PROGRAM P_Prog3
VAR

	fbKL6401 					: FB_LON_KL6401;

	fbREAD_063		: FB_READ_063_SNVT_temp_f;
	fbSEND_063		: FB_SEND_063_SNVT_temp_f;

	fbREAD_064		: FB_READ_064_SNVT_time_f;
	fbSEND_064		: FB_SEND_064_SNVT_time_f;

	fbREAD_065		: FB_READ_065_SNVT_vol_f;
	fbSEND_065		: FB_SEND_065_SNVT_vol_f;

	fbREAD_066		: FB_READ_066_SNVT_volt_f;
	fbSEND_066		: FB_SEND_066_SNVT_volt_f;

	fbREAD_067		: FB_READ_067_SNVT_btu_f;
	fbSEND_067		: FB_SEND_067_SNVT_btu_f;

	fbREAD_068		: FB_READ_068_SNVT_elec_whr_f;
	fbSEND_068		: FB_SEND_068_SNVT_elec_whr_f;

	fbREAD_069		: FB_READ_069_SNVT_config_src;
	fbSEND_069		: FB_SEND_069_SNVT_config_src;

	fbREAD_070		: FB_READ_070_SNVT_color;
	fbSEND_070		: FB_SEND_070_SNVT_color;

	fbREAD_071		: FB_READ_071_SNVT_grammage;
	fbSEND_071		: FB_SEND_071_SNVT_grammage;

	fbREAD_072		: FB_READ_072_SNVT_grammage_f;
	fbSEND_072		: FB_SEND_072_SNVT_grammage_f;

	fbREAD_073		: FB_READ_073_SNVT_file_req;
	fbSEND_073		: FB_SEND_073_SNVT_file_req;

	fbREAD_074		: FB_READ_074_SNVT_file_status;
	fbSEND_074		: FB_SEND_074_SNVT_file_status;

	fbREAD_075		: FB_READ_075_SNVT_freq_f;
	fbSEND_075		: FB_SEND_075_SNVT_freq_f;

	fbREAD_076		: FB_READ_076_SNVT_freq_hz;
	fbSEND_076		: FB_SEND_076_SNVT_freq_hz;

	fbREAD_077		: FB_READ_077_SNVT_freq_kilohz;
	fbSEND_077		: FB_SEND_077_SNVT_freq_kilohz;

	fbREAD_078		: FB_READ_078_SNVT_freq_milhz;
	fbSEND_078		: FB_SEND_078_SNVT_freq_milhz;

	fbREAD_079		: FB_READ_079_SNVT_lux;
	fbSEND_079		: FB_SEND_079_SNVT_lux;
(*
	fbREAD_080		: FB_READ_080;
	fbSEND_080		: FB_SEND_080_SNVT_angle_vel_f;
*)
	fbREAD_081		: FB_READ_081_SNVT_lev_percent;
	fbSEND_081		: FB_SEND_081_SNVT_lev_percent;

	fbREAD_082		: FB_READ_082_SNVT_multiplier;
	fbSEND_082		: FB_SEND_082_SNVT_multiplier;

	fbREAD_083		: FB_READ_083_SNVT_state;
	fbSEND_083		: FB_SEND_083_SNVT_state;

	fbREAD_084		: FB_READ_084_SNVT_time_stamp;
	fbSEND_084		: FB_SEND_084_SNVT_time_stamp;

	fbREAD_085		: FB_READ_085_SNVT_zerospan;
	fbSEND_085		: FB_SEND_085_SNVT_zerospan;

	fbREAD_086		: FB_READ_086_SNVT_magcard;
	fbSEND_086		: FB_SEND_086_SNVT_magcard;

	fbREAD_087		: FB_READ_087_SNVT_elapsed_tm;
	fbSEND_087		: FB_SEND_087_SNVT_elapsed_tm;

	fbREAD_088		: FB_READ_088_SNVT_alarm;
	fbSEND_088		: FB_SEND_088_SNVT_alarm;

	fbREAD_089		: FB_READ_089_SNVT_currency;
	fbSEND_089		: FB_SEND_089_SNVT_currency;

	fbREAD_090		: FB_READ_090_SNVT_file_pos;
	fbSEND_090		: FB_SEND_090_SNVT_file_pos;

	fbREAD_091		: FB_READ_091_SNVT_muldiv;
	fbSEND_091		: FB_SEND_091_SNVT_muldiv;

	fbREAD_092		: FB_READ_092_SNVT_obj_request;
	fbSEND_092		: FB_SEND_092_SNVT_obj_request;

	fbREAD_093		: FB_READ_093_SNVT_obj_status;
	fbSEND_093		: FB_SEND_093_SNVT_obj_status;

END_VAR


fbKL6401(
	bDisabled:=FALSE ,
	stParameter_IN:=LON_IN_3 ,
	stParameter_OUT:=LON_OUT_3 ,
	stLON_Com:=stLON_Com_3,
	bReady=> ,
	eError=> ,
	stKL6401=> ,
	arrProgID=> ,
	arrNeuronID=> ,
	bBusy=> ,
	bError=> ,
	dwErrorKL=> ,
	bTimeOut=> ,
	byLONState=> );

(**)
fbREAD_063(
	wNVIndex:=0 ,
	bDisabled:= ,
	stLON_Com:=stLON_Com_3,
	rValue=> ,
	bNewData=> ,
	bError=> ,
	eError=> );
fbREAD_063.rValue;
fbREAD_063.bError;
fbREAD_063.eError;

fbSEND_063.rValue;
fbSEND_063.bStart;
fbSEND_063.bError;
fbSEND_063.eError;
fbSEND_063.bBusy;
fbSEND_063.dwErrorKL;

fbSEND_063.bAuto;
fbSEND_063.bSendInit;
fbSEND_063.tMinSendTime;
fbSEND_063.tMaxSendTime;
fbSEND_063.rValueLimit;

fbSEND_063(
	wNVIndex:=1 ,
	bStart:= ,
	rValue:= ,
	bDisabled:= ,
	stLON_Com:=stLON_Com_3,
	bError=> ,
	eError=> );
fbSEND_063.bStart:=FALSE;

(**)
fbREAD_064(
	wNVIndex:=2 ,
	bDisabled:= ,
	stLON_Com:=stLON_Com_3,
	rValue=> ,
	bNewData=> ,
	bError=> ,
	eError=> );
fbREAD_064.rValue;
fbREAD_064.bError;
fbREAD_064.eError;

fbSEND_064.rValue;
fbSEND_064.bStart;
fbSEND_064.bError;
fbSEND_064.eError;
fbSEND_064.bBusy;
fbSEND_064.dwErrorKL;

fbSEND_064.bAuto;
fbSEND_064.bSendInit;
fbSEND_064.tMinSendTime;
fbSEND_064.tMaxSendTime;
fbSEND_064.rValueLimit;

fbSEND_064(
	wNVIndex:=3 ,
	bStart:= ,
	rValue:= ,
	bDisabled:= ,
	stLON_Com:=stLON_Com_3,
	bError=> ,
	eError=> );
fbSEND_064.bStart:=FALSE;

(**)
fbREAD_065(
	wNVIndex:=4 ,
	bDisabled:= ,
	stLON_Com:=stLON_Com_3,
	rValue=> ,
	bNewData=> ,
	bError=> ,
	eError=> );
fbREAD_065.rValue;
fbREAD_065.bError;
fbREAD_065.eError;

fbSEND_065.rValue;
fbSEND_065.bStart;
fbSEND_065.bError;
fbSEND_065.eError;
fbSEND_065.bBusy;
fbSEND_065.dwErrorKL;

fbSEND_065.bAuto;
fbSEND_065.bSendInit;
fbSEND_065.tMinSendTime;
fbSEND_065.tMaxSendTime;
fbSEND_065.rValueLimit;

fbSEND_065(
	wNVIndex:=5 ,
	bStart:= ,
	rValue:= ,
	bDisabled:= ,
	stLON_Com:=stLON_Com_3,
	bError=> ,
	eError=> );
fbSEND_065.bStart:=FALSE;

(**)
fbREAD_066(
	wNVIndex:=6 ,
	bDisabled:= ,
	stLON_Com:=stLON_Com_3,
	rValue=> ,
	bNewData=> ,
	bError=> ,
	eError=> );
fbREAD_066.rValue;
fbREAD_066.bError;
fbREAD_066.eError;

fbSEND_066.rValue;
fbSEND_066.bStart;
fbSEND_066.bError;
fbSEND_066.eError;
fbSEND_066.bBusy;
fbSEND_066.dwErrorKL;

fbSEND_066.bAuto;
fbSEND_066.bSendInit;
fbSEND_066.tMinSendTime;
fbSEND_066.tMaxSendTime;
fbSEND_066.rValueLimit;

fbSEND_066(
	wNVIndex:=7 ,
	bStart:= ,
	rValue:= ,
	bDisabled:= ,
	stLON_Com:=stLON_Com_3,
	bError=> ,
	eError=> );
fbSEND_066.bStart:=FALSE;

(**)
fbREAD_067(
	wNVIndex:=8 ,
	bDisabled:= ,
	stLON_Com:=stLON_Com_3,
	rValue=> ,
	bNewData=> ,
	bError=> ,
	eError=> );
fbREAD_067.rValue;
fbREAD_067.bError;
fbREAD_067.eError;

fbSEND_067.rValue;
fbSEND_067.bStart;
fbSEND_067.bError;
fbSEND_067.eError;
fbSEND_067.bBusy;
fbSEND_067.dwErrorKL;

fbSEND_067.bAuto;
fbSEND_067.bSendInit;
fbSEND_067.tMinSendTime;
fbSEND_067.tMaxSendTime;
fbSEND_067.rValueLimit;

fbSEND_067(
	wNVIndex:=9 ,
	bStart:= ,
	rValue:= ,
	bDisabled:= ,
	stLON_Com:=stLON_Com_3,
	bError=> ,
	eError=> );
fbSEND_067.bStart:=FALSE;

(**)
fbREAD_068(
	wNVIndex:=10 ,
	bDisabled:= ,
	stLON_Com:=stLON_Com_3,
	rValue=> ,
	bNewData=> ,
	bError=> ,
	eError=> );
fbREAD_068.rValue;
fbREAD_068.bError;
fbREAD_068.eError;

fbSEND_068.rValue;
fbSEND_068.bStart;
fbSEND_068.bError;
fbSEND_068.eError;
fbSEND_068.bBusy;
fbSEND_068.dwErrorKL;

fbSEND_068.bAuto;
fbSEND_068.bSendInit;
fbSEND_068.tMinSendTime;
fbSEND_068.tMaxSendTime;
fbSEND_068.rValueLimit;

fbSEND_068(
	wNVIndex:=11 ,
	bStart:= ,
	rValue:= ,
	bDisabled:= ,
	stLON_Com:=stLON_Com_3,
	bError=> ,
	eError=> );
fbSEND_068.bStart:=FALSE;

(**)
fbREAD_069(
	wNVIndex:=12 ,
	bDisabled:= ,
	stLON_Com:=stLON_Com_3,
	eValue=> ,
	bNewData=> ,
	bError=> ,
	eError=> );
fbREAD_069.eValue;
fbREAD_069.bError;
fbREAD_069.eError;

fbSEND_069.eValue;
fbSEND_069.bStart;
fbSEND_069.bError;
fbSEND_069.eError;
fbSEND_069.bBusy;
fbSEND_069.dwErrorKL;

fbSEND_069.bAuto;
fbSEND_069.bSendInit;
fbSEND_069.tMinSendTime;
fbSEND_069.tMaxSendTime;

fbSEND_069(
	wNVIndex:=13 ,
	bStart:= ,
	eValue:= ,
	bDisabled:= ,
	stLON_Com:=stLON_Com_3,
	bError=> ,
	eError=> );
fbSEND_069.bStart:=FALSE;

(**)
fbREAD_070(
	wNVIndex:=14 ,
	bDisabled:= ,
	stLON_Com:=stLON_Com_3,
	stValue=> ,
	bNewData=> ,
	bError=> ,
	eError=> );
fbREAD_070.stValue;
fbREAD_070.bError;
fbREAD_070.eError;

fbSEND_070.stValue;
fbSEND_070.bStart;
fbSEND_070.bError;
fbSEND_070.eError;
fbSEND_070.bBusy;
fbSEND_070.dwErrorKL;

fbSEND_070.bAuto;
fbSEND_070.bSendInit;
fbSEND_070.tMinSendTime;
fbSEND_070.tMaxSendTime;

fbSEND_070(
	wNVIndex:=15 ,
	bStart:= ,
	stValue:= ,
	bDisabled:= ,
	stLON_Com:=stLON_Com_3,
	bError=> ,
	eError=> );
fbSEND_070.bStart:=FALSE;

(**)
fbREAD_071(
	wNVIndex:=16 ,
	bDisabled:= ,
	stLON_Com:=stLON_Com_3,
	rValue=> ,
	bNewData=> ,
	bError=> ,
	eError=> );
fbREAD_071.rValue;
fbREAD_071.bError;
fbREAD_071.eError;

fbSEND_071.rValue;
fbSEND_071.bStart;
fbSEND_071.bError;
fbSEND_071.eError;
fbSEND_071.bBusy;
fbSEND_071.dwErrorKL;

fbSEND_071.bAuto;
fbSEND_071.bSendInit;
fbSEND_071.tMinSendTime;
fbSEND_071.tMaxSendTime;
fbSEND_071.rValueLimit;

fbSEND_071(
	wNVIndex:=17 ,
	bStart:= ,
	rValue:= ,
	bDisabled:= ,
	stLON_Com:=stLON_Com_3,
	bError=> ,
	eError=> );
fbSEND_071.bStart:=FALSE;

(**)
fbREAD_072(
	wNVIndex:=18 ,
	bDisabled:= ,
	stLON_Com:=stLON_Com_3,
	rValue=> ,
	bNewData=> ,
	bError=> ,
	eError=> );
fbREAD_072.rValue;
fbREAD_072.bError;
fbREAD_072.eError;

fbSEND_072.rValue;
fbSEND_072.bStart;
fbSEND_072.bError;
fbSEND_072.eError;
fbSEND_072.bBusy;
fbSEND_072.dwErrorKL;

fbSEND_072.bAuto;
fbSEND_072.bSendInit;
fbSEND_072.tMinSendTime;
fbSEND_072.tMaxSendTime;
fbSEND_072.rValueLimit;

fbSEND_072(
	wNVIndex:=19 ,
	bStart:= ,
	rValue:= ,
	bDisabled:= ,
	stLON_Com:=stLON_Com_3,
	bError=> ,
	eError=> );
fbSEND_072.bStart:=FALSE;

(**)
fbREAD_073(
	wNVIndex:=20 ,
	bDisabled:= ,
	stLON_Com:=stLON_Com_3,
	stValue=> ,
	bNewData=> ,
	bError=> ,
	eError=> );
fbREAD_073.stValue;
fbREAD_073.bError;
fbREAD_073.eError;

fbSEND_073.stValue;
fbSEND_073.bStart;
fbSEND_073.bError;
fbSEND_073.eError;
fbSEND_073.bBusy;
fbSEND_073.dwErrorKL;

fbSEND_073.bAuto;
fbSEND_073.bSendInit;
fbSEND_073.tMinSendTime;
fbSEND_073.tMaxSendTime;

fbSEND_073(
	wNVIndex:=21 ,
	bStart:= ,
	stValue:= ,
	bDisabled:= ,
	stLON_Com:=stLON_Com_3,
	bError=> ,
	eError=> );
fbSEND_073.bStart:=FALSE;

(**)
fbREAD_074(
	wNVIndex:=22 ,
	bDisabled:= ,
	stLON_Com:=stLON_Com_3,
	stValue=> ,
	bNewData=> ,
	bError=> ,
	eError=> );
fbREAD_074.stValue;
fbREAD_074.bError;
fbREAD_074.eError;

fbSEND_074.stValue;
fbSEND_074.bStart;
fbSEND_074.bError;
fbSEND_074.eError;
fbSEND_074.bBusy;
fbSEND_074.dwErrorKL;

fbSEND_074.bAuto;
fbSEND_074.bSendInit;
fbSEND_074.tMinSendTime;
fbSEND_074.tMaxSendTime;

fbSEND_074(
	wNVIndex:=23 ,
	bStart:= ,
	stValue:= ,
	bDisabled:= ,
	stLON_Com:=stLON_Com_3,
	bError=> ,
	eError=> );
fbSEND_074.bStart:=FALSE;

(**)
fbREAD_075(
	wNVIndex:=24 ,
	bDisabled:= ,
	stLON_Com:=stLON_Com_3,
	rValue=> ,
	bNewData=> ,
	bError=> ,
	eError=> );
fbREAD_075.rValue;
fbREAD_075.bError;
fbREAD_075.eError;

fbSEND_075.rValue;
fbSEND_075.bStart;
fbSEND_075.bError;
fbSEND_075.eError;
fbSEND_075.bBusy;
fbSEND_075.dwErrorKL;

fbSEND_075.bAuto;
fbSEND_075.bSendInit;
fbSEND_075.tMinSendTime;
fbSEND_075.tMaxSendTime;
fbSEND_075.rValueLimit;

fbSEND_075(
	wNVIndex:=25 ,
	bStart:= ,
	rValue:= ,
	bDisabled:= ,
	stLON_Com:=stLON_Com_3,
	bError=> ,
	eError=> );
fbSEND_075.bStart:=FALSE;

(**)
fbREAD_076(
	wNVIndex:=26 ,
	bDisabled:= ,
	stLON_Com:=stLON_Com_3,
	rValue=> ,
	bNewData=> ,
	bError=> ,
	eError=> );
fbREAD_076.rValue;
fbREAD_076.bError;
fbREAD_076.eError;

fbSEND_076.rValue;
fbSEND_076.bStart;
fbSEND_076.bError;
fbSEND_076.eError;
fbSEND_076.bBusy;
fbSEND_076.dwErrorKL;

fbSEND_076.bAuto;
fbSEND_076.bSendInit;
fbSEND_076.tMinSendTime;
fbSEND_076.tMaxSendTime;
fbSEND_076.rValueLimit;

fbSEND_076(
	wNVIndex:=27 ,
	bStart:= ,
	rValue:= ,
	bDisabled:= ,
	stLON_Com:=stLON_Com_3,
	bError=> ,
	eError=> );
fbSEND_076.bStart:=FALSE;

(**)
fbREAD_077(
	wNVIndex:=28 ,
	bDisabled:= ,
	stLON_Com:=stLON_Com_3,
	rValue=> ,
	bNewData=> ,
	bError=> ,
	eError=> );
fbREAD_077.rValue;
fbREAD_077.bError;
fbREAD_077.eError;

fbSEND_077.rValue;
fbSEND_077.bStart;
fbSEND_077.bError;
fbSEND_077.eError;
fbSEND_077.bBusy;
fbSEND_077.dwErrorKL;

fbSEND_077.bAuto;
fbSEND_077.bSendInit;
fbSEND_077.tMinSendTime;
fbSEND_077.tMaxSendTime;
fbSEND_077.rValueLimit;

fbSEND_077(
	wNVIndex:=29 ,
	bStart:= ,
	rValue:= ,
	bDisabled:= ,
	stLON_Com:=stLON_Com_3,
	bError=> ,
	eError=> );
fbSEND_077.bStart:=FALSE;

(**)
fbREAD_078(
	wNVIndex:=30 ,
	bDisabled:= ,
	stLON_Com:=stLON_Com_3,
	rValue=> ,
	bNewData=> ,
	bError=> ,
	eError=> );
fbREAD_078.rValue;
fbREAD_078.bError;
fbREAD_078.eError;

fbSEND_078.rValue;
fbSEND_078.bStart;
fbSEND_078.bError;
fbSEND_078.eError;
fbSEND_078.bBusy;
fbSEND_078.dwErrorKL;

fbSEND_078.bAuto;
fbSEND_078.bSendInit;
fbSEND_078.tMinSendTime;
fbSEND_078.tMaxSendTime;
fbSEND_078.rValueLimit;

fbSEND_078(
	wNVIndex:=31 ,
	bStart:= ,
	rValue:= ,
	bDisabled:= ,
	stLON_Com:=stLON_Com_3,
	bError=> ,
	eError=> );
fbSEND_078.bStart:=FALSE;

(**)
fbREAD_079(
	wNVIndex:=32 ,
	bDisabled:= ,
	stLON_Com:=stLON_Com_3,
	uiValue=> ,
	bNewData=> ,
	bError=> ,
	eError=> );
fbREAD_079.uiValue;
fbREAD_079.bError;
fbREAD_079.eError;

fbSEND_079.uiValue;
fbSEND_079.bStart;
fbSEND_079.bError;
fbSEND_079.eError;
fbSEND_079.bBusy;
fbSEND_079.dwErrorKL;

fbSEND_079.bAuto;
fbSEND_079.bSendInit;
fbSEND_079.tMinSendTime;
fbSEND_079.tMaxSendTime;
fbSEND_079.uiValueLimit;

fbSEND_079(
	wNVIndex:=33 ,
	bStart:= ,
	uiValue:= ,
	bDisabled:= ,
	stLON_Com:=stLON_Com_3,
	bError=> ,
	eError=> );
fbSEND_079.bStart:=FALSE;

(**)
(*
fbREAD_080(
	wNVIndex:=34 ,
	bDisabled:= ,
	stLON_Com:=stLON_Com_3,
	rValue=> ,
	bNewData=> ,
	bError=> ,
	eError=> );
fbREAD_080.rValue;
fbREAD_080.bError;
fbREAD_080.eError;

fbSEND_080(
	wNVIndex:=35 ,
	bStart:= ,
	rValue:= ,
	bDisabled:= ,
	stLON_Com:=stLON_Com_3,
	bError=> ,
	eError=> );
fbSEND_080.rValue;
fbSEND_080.bStart;
fbSEND_080.bError;
fbSEND_080.eError;
*)

(**)
fbREAD_081(
	wNVIndex:=36 ,
	bDisabled:= ,
	stLON_Com:=stLON_Com_3,
	rValue=> ,
	bNewData=> ,
	bError=> ,
	eError=> );
fbREAD_081.rValue;
fbREAD_081.bError;
fbREAD_081.eError;

fbSEND_081.rValue;
fbSEND_081.bStart;
fbSEND_081.bError;
fbSEND_081.eError;
fbSEND_081.bBusy;
fbSEND_081.dwErrorKL;

fbSEND_081.bAuto;
fbSEND_081.bSendInit;
fbSEND_081.tMinSendTime;
fbSEND_081.tMaxSendTime;
fbSEND_081.rValueLimit;

fbSEND_081(
	wNVIndex:=37 ,
	bStart:= ,
	rValue:= ,
	bDisabled:= ,
	stLON_Com:=stLON_Com_3,
	bError=> ,
	eError=> );
fbSEND_081.bStart:=FALSE;

(**)
fbREAD_082(
	wNVIndex:=38 ,
	bDisabled:= ,
	stLON_Com:=stLON_Com_3,
	rValue=> ,
	bNewData=> ,
	bError=> ,
	eError=> );
fbREAD_082.rValue;
fbREAD_082.bError;
fbREAD_082.eError;

fbSEND_082.rValue;
fbSEND_082.bStart;
fbSEND_082.bError;
fbSEND_082.eError;
fbSEND_082.bBusy;
fbSEND_082.dwErrorKL;

fbSEND_082.bAuto;
fbSEND_082.bSendInit;
fbSEND_082.tMinSendTime;
fbSEND_082.tMaxSendTime;
fbSEND_082.rValueLimit;

fbSEND_082(
	wNVIndex:=39 ,
	bStart:= ,
	rValue:= ,
	bDisabled:= ,
	stLON_Com:=stLON_Com_3,
	bError=> ,
	eError=> );
fbSEND_082.bStart:=FALSE;

(**)
fbREAD_083(
	wNVIndex:=40 ,
	bDisabled:= ,
	stLON_Com:=stLON_Com_3,
	arrValue=> ,
	bNewData=> ,
	bError=> ,
	eError=> );
fbREAD_083.arrValue;
fbREAD_083.bError;
fbREAD_083.eError;

fbSEND_083.arrValue;
fbSEND_083.bStart;
fbSEND_083.bError;
fbSEND_083.eError;
fbSEND_083.bBusy;
fbSEND_083.dwErrorKL;

fbSEND_083.bAuto;
fbSEND_083.bSendInit;
fbSEND_083.tMinSendTime;
fbSEND_083.tMaxSendTime;

fbSEND_083(
	wNVIndex:=41 ,
	bStart:= ,
	arrValue:= ,
	bDisabled:= ,
	stLON_Com:=stLON_Com_3,
	bError=> ,
	eError=> );
fbSEND_083.bStart:=FALSE;

(**)
fbREAD_084(
	wNVIndex:=42 ,
	bDisabled:= ,
	stLON_Com:=stLON_Com_3,
	stValue=> ,
	bNewData=> ,
	bError=> ,
	eError=> );
fbREAD_084.stValue;
fbREAD_084.bError;
fbREAD_084.eError;

fbSEND_084.stValue;
fbSEND_084.bStart;
fbSEND_084.bError;
fbSEND_084.eError;
fbSEND_084.bBusy;
fbSEND_084.dwErrorKL;

fbSEND_084.bAuto;
fbSEND_084.bSendInit;
fbSEND_084.tMinSendTime;
fbSEND_084.tMaxSendTime;

fbSEND_084(
	wNVIndex:=43 ,
	bStart:= ,
	stValue:= ,
	bDisabled:= ,
	stLON_Com:=stLON_Com_3,
	bError=> ,
	eError=> );
fbSEND_084.bStart:=FALSE;

(**)
fbREAD_085(
	wNVIndex:=44 ,
	bDisabled:= ,
	stLON_Com:=stLON_Com_3,
	stValue=> ,
	bNewData=> ,
	bError=> ,
	eError=> );
fbREAD_085.stValue;
fbREAD_085.bError;
fbREAD_085.eError;

fbSEND_085.stValue;
fbSEND_085.bStart;
fbSEND_085.bError;
fbSEND_085.eError;
fbSEND_085.bBusy;
fbSEND_085.dwErrorKL;

fbSEND_085.bAuto;
fbSEND_085.bSendInit;
fbSEND_085.tMinSendTime;
fbSEND_085.tMaxSendTime;

fbSEND_085(
	wNVIndex:=45 ,
	bStart:= ,
	stValue:= ,
	bDisabled:= ,
	stLON_Com:=stLON_Com_3,
	bError=> ,
	eError=> );
fbSEND_085.bStart:=FALSE;

(**)
fbREAD_086(
	wNVIndex:=46 ,
	bDisabled:= ,
	stLON_Com:=stLON_Com_3,
	arrValue=> ,
	bNewData=> ,
	bError=> ,
	eError=> );
fbREAD_086.arrValue;
fbREAD_086.bError;
fbREAD_086.eError;
fbSEND_086.bBusy;
fbSEND_086.dwErrorKL;

fbSEND_086.arrValue;
fbSEND_086.bStart;
fbSEND_086.bError;
fbSEND_086.eError;

fbSEND_086.bAuto;
fbSEND_086.bSendInit;
fbSEND_086.tMinSendTime;
fbSEND_086.tMaxSendTime;

fbSEND_086(
	wNVIndex:=47 ,
	bStart:= ,
	arrValue:= ,
	bDisabled:= ,
	stLON_Com:=stLON_Com_3,
	bError=> ,
	eError=> );
fbSEND_086.bStart:=FALSE;

(**)
fbREAD_087(
	wNVIndex:=48 ,
	bDisabled:= ,
	stLON_Com:=stLON_Com_3,
	stValue=> ,
	bNewData=> ,
	bError=> ,
	eError=> );
fbREAD_087.stValue;
fbREAD_087.bError;
fbREAD_087.eError;

fbSEND_087.stValue;
fbSEND_087.bStart;
fbSEND_087.bError;
fbSEND_087.eError;
fbSEND_087.bBusy;
fbSEND_087.dwErrorKL;

fbSEND_087.bAuto;
fbSEND_087.bSendInit;
fbSEND_087.tMinSendTime;
fbSEND_087.tMaxSendTime;

fbSEND_087(
	wNVIndex:=49 ,
	bStart:= ,
	stValue:= ,
	bDisabled:= ,
	stLON_Com:=stLON_Com_3,
	bError=> ,
	eError=> );
fbSEND_087.bStart:=FALSE;

(**)
fbREAD_088(
	wNVIndex:=50 ,
	bDisabled:= ,
	stLON_Com:=stLON_Com_3,
	stValue=> ,
	bNewData=> ,
	bError=> ,
	eError=> );
fbREAD_088.stValue;
fbREAD_088.bError;
fbREAD_088.eError;

fbSEND_088.stValue;
fbSEND_088.bStart;
fbSEND_088.bError;
fbSEND_088.eError;
fbSEND_088.bBusy;
fbSEND_088.dwErrorKL;

fbSEND_088.bAuto;
fbSEND_088.bSendInit;
fbSEND_088.tMinSendTime;
fbSEND_088.tMaxSendTime;

fbSEND_088(
	wNVIndex:=51 ,
	bStart:= ,
	stValue:= ,
	bDisabled:= ,
	stLON_Com:=stLON_Com_3,
	bError=> ,
	eError=> );
fbSEND_088.bStart:=FALSE;

(**)
fbREAD_089(
	wNVIndex:=52 ,
	bDisabled:= ,
	stLON_Com:=stLON_Com_3,
	stValue=> ,
	bNewData=> ,
	bError=> ,
	eError=> );
fbREAD_089.stValue;
fbREAD_089.bError;
fbREAD_089.eError;

fbSEND_089.stValue;
fbSEND_089.bStart;
fbSEND_089.bError;
fbSEND_089.eError;
fbSEND_089.bBusy;
fbSEND_089.dwErrorKL;

fbSEND_089.bAuto;
fbSEND_089.bSendInit;
fbSEND_089.tMinSendTime;
fbSEND_089.tMaxSendTime;

fbSEND_089(
	wNVIndex:=53 ,
	bStart:= ,
	stValue:= ,
	bDisabled:= ,
	stLON_Com:=stLON_Com_3,
	bError=> ,
	eError=> );
fbSEND_089.bStart:=FALSE;

(**)
fbREAD_090(
	wNVIndex:=54 ,
	bDisabled:= ,
	stLON_Com:=stLON_Com_3,
	stValue=> ,
	bNewData=> ,
	bError=> ,
	eError=> );
fbREAD_090.stValue;
fbREAD_090.bError;
fbREAD_090.eError;

fbSEND_090.stValue;
fbSEND_090.bStart;
fbSEND_090.bError;
fbSEND_090.eError;
fbSEND_090.bBusy;
fbSEND_090.dwErrorKL;

fbSEND_090.bAuto;
fbSEND_090.bSendInit;
fbSEND_090.tMinSendTime;
fbSEND_090.tMaxSendTime;

fbSEND_090(
	wNVIndex:=55 ,
	bStart:= ,
	stValue:= ,
	bDisabled:= ,
	stLON_Com:=stLON_Com_3,
	bError=> ,
	eError=> );
fbSEND_090.bStart:=FALSE;

(**)
fbREAD_091(
	wNVIndex:=56 ,
	bDisabled:= ,
	stLON_Com:=stLON_Com_3,
	stValue=> ,
	bNewData=> ,
	bError=> ,
	eError=> );
fbREAD_091.stValue;
fbREAD_091.bError;
fbREAD_091.eError;

fbSEND_091.stValue;
fbSEND_091.bStart;
fbSEND_091.bError;
fbSEND_091.eError;
fbSEND_091.bBusy;
fbSEND_091.dwErrorKL;

fbSEND_091.bAuto;
fbSEND_091.bSendInit;
fbSEND_091.tMinSendTime;
fbSEND_091.tMaxSendTime;

fbSEND_091(
	wNVIndex:=57 ,
	bStart:= ,
	stValue:= ,
	bDisabled:= ,
	stLON_Com:=stLON_Com_3,
	bError=> ,
	eError=> );
fbSEND_091.bStart:=FALSE;

(**)
fbREAD_092(
	wNVIndex:=58 ,
	bDisabled:= ,
	stLON_Com:=stLON_Com_3,
	stValue=> ,
	bNewData=> ,
	bError=> ,
	eError=> );
fbREAD_092.stValue;
fbREAD_092.bError;
fbREAD_092.eError;

fbSEND_092.stValue;
fbSEND_092.bStart;
fbSEND_092.bError;
fbSEND_092.eError;
fbSEND_092.bBusy;
fbSEND_092.dwErrorKL;

fbSEND_092.bAuto;
fbSEND_092.bSendInit;
fbSEND_092.tMinSendTime;
fbSEND_092.tMaxSendTime;

fbSEND_092(
	wNVIndex:=59 ,
	bStart:= ,
	stValue:= ,
	bDisabled:= ,
	stLON_Com:=stLON_Com_3,
	bError=> ,
	eError=> );
fbSEND_092.bStart:=FALSE;

(**)
fbREAD_093(
	wNVIndex:=60 ,
	bDisabled:= ,
	stLON_Com:=stLON_Com_3,
	stValue=> ,
	bNewData=> ,
	bError=> ,
	eError=> );
fbREAD_093.stValue;
fbREAD_093.bError;
fbREAD_093.eError;

fbSEND_093.stValue;
fbSEND_093.bStart;
fbSEND_093.bError;
fbSEND_093.eError;
fbSEND_093.bBusy;
fbSEND_093.dwErrorKL;

fbSEND_093.bAuto;
fbSEND_093.bSendInit;
fbSEND_093.tMinSendTime;
fbSEND_093.tMaxSendTime;

fbSEND_093(
	wNVIndex:=61 ,
	bStart:= ,
	stValue:= ,
	bDisabled:= ,
	stLON_Com:=stLON_Com_3,
	bError=> ,
	eError=> );
fbSEND_093.bStart:=FALSE;

END_PROGRAM
